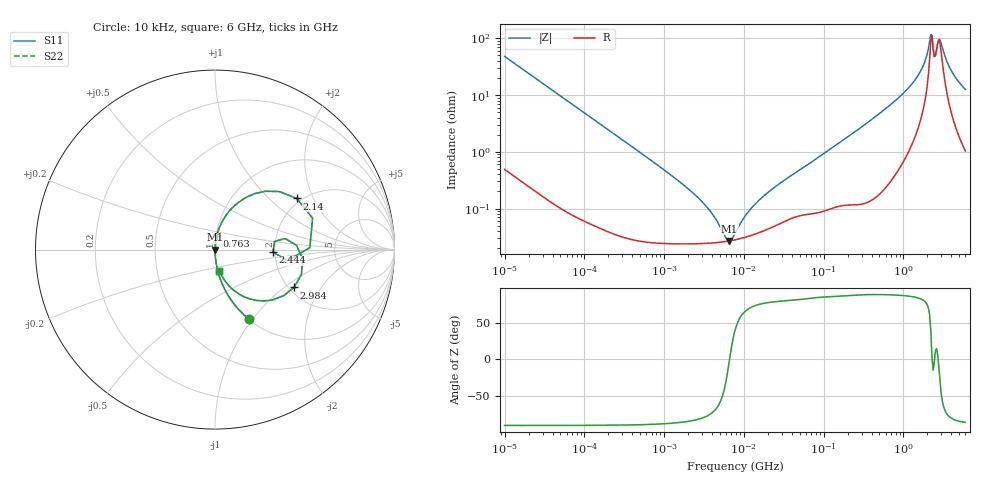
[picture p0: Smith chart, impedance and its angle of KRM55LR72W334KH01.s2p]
!Murata Part Number: KRM55LR72W334KH01
!These Parameters are Measured in Series Mode Connection
!Data Generated on Jan 08, 2026
!  o--ll--o
!Port1  Port2
!  o------o
!Operation Temp=25[degC], DC Bias Voltage=0[V]
!Freq. Start=10[kHz] Stop=6[GHz] 401[Steps]
# Hz S RI R 50
!Freq.(Hz) S11(Real) S11(Imag) S21(Real) S21(Imag) S12(Real) S12(Imag) S22(Real) S22(Imag)
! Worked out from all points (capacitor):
!   401 points, 10 kHz to 6 GHz, reference 50 ohm
!   read as one part in series: C = 331 nF near 10.69 kHz
!   lowest |Z| = 26.8 mohm at 6.559 MHz (marker M1)
!   series resonance near 6.616 MHz, so ESL is about 1.7 nH
!   S11 on the Smith chart (normalised r, x): 10 kHz: 1.01, -0.96; 763 MHz: 1.01, +0.15; 2.14 GHz: 1.88, +1.51; 2.444 GHz: 1.95, -0.06; 2.984 GHz: 2.13, -1.18; 6 GHz: 1.02, -0.25
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10000  0.1893 -0.3867  0.8107 0.3867  0.8107 0.3867  0.1893 -0.3867
22969  0.044 -0.2001  0.956 0.2001  0.956 0.2001  0.044 -0.2001
92862  0.00334 -0.052  0.9967 0.052  0.9967 0.052  0.00334 -0.052
862344  0.000275 -0.00557  0.9997 0.00557  0.9997 0.00557  0.000275 -0.00557
3052144  0.000243 -0.00126  0.9998 0.00126  0.9998 0.00126  0.000243 -0.00126
6559168  0.000268 -1.25e-05  0.9997 1.25e-05  0.9997 1.25e-05  0.000268 -1.25e-05
7745967  0.00028 0.00023  0.9997 -0.00023  0.9997 -0.00023  0.00028 0.00023
1.044922e7  0.000312 0.000679  0.9997 -0.000679  0.9997 -0.000679  0.000312 0.000679
1.557502e7  0.000377 0.00136  0.9996 -0.00136  0.9996 -0.00136  0.000377 0.00136
7.193098e7  0.000851 0.00666  0.9991 -0.00666  0.9991 -0.00666  0.000851 0.00666
6.67969e8  0.00697 0.0644  0.993 -0.0644  0.993 -0.0644  0.00697 0.0644
7.630233e8  0.00929 0.0751  0.9907 -0.0751  0.9907 -0.0751  0.00929 0.0751
1.215551e9  0.0307 0.1374  0.9693 -0.1374  0.9693 -0.1374  0.0307 0.1374
1.639765e9  0.0911 0.2271  0.9089 -0.2271  0.9089 -0.2271  0.0911 0.2271
2.001953e9  0.2806 0.3251  0.7194 -0.3251  0.7194 -0.3251  0.2806 0.3251
2.139659e9  0.4562 0.2852  0.5438 -0.2852  0.5438 -0.2852  0.4562 0.2852
2.44414e9  0.3227 -0.0144  0.6773 0.0144  0.6773 0.0144  0.3227 -0.0144
2.700612e9  0.454 0.024  0.546 -0.024  0.546 -0.024  0.454 0.024
2.983997e9  0.4399 -0.2109  0.5601 0.2109  0.5601 0.2109  0.4399 -0.2109
3.297118e9  0.2702 -0.2863  0.7298 0.2863  0.7298 0.2863  0.2702 -0.2863
3.89369e9  0.1156 -0.2354  0.8844 0.2354  0.8844 0.2354  0.1156 -0.2354
6e9  0.0251 -0.1204  0.9749 0.1204  0.9749 0.1204  0.0251 -0.1204
